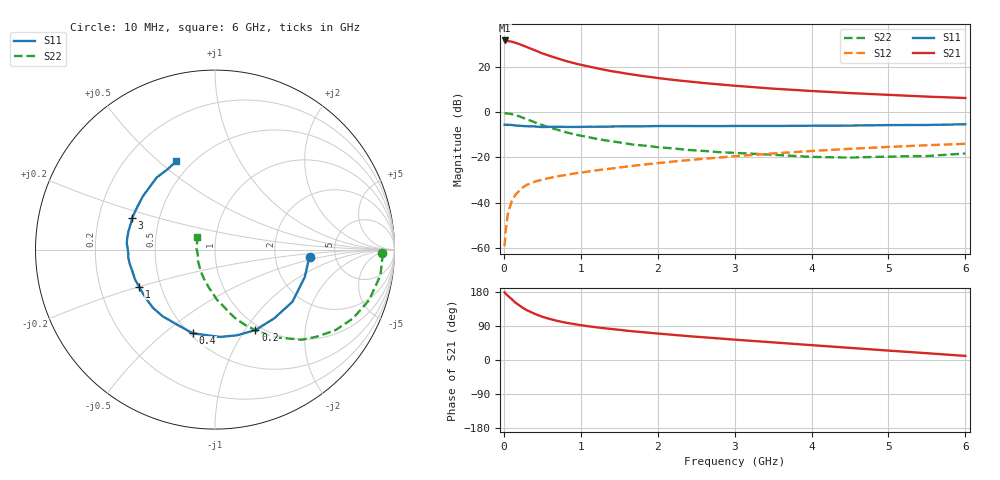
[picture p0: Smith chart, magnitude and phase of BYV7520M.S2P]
! SIEMENS Small Signal Semiconductors
! BFY420
! Si NPN RF SIEGET Grounded Emitter Transistor in MICRO-X
! VCE = 0.75 V  IC = 20 mA
! Common Emitter S-Parameters:  October  1996
# GHz  S  MA  R  50
!  f  S11  S21  S12  S22
! GHz  MAG  ANG  MAG  ANG  MAG  ANG  MAG  ANG
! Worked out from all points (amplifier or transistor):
!   36 points, 10 MHz to 6 GHz, reference 50 ohm
!   highest |S21| = 31.6 dB at 10 MHz (marker M1)
!   |S21| within 3 dB of that: start of sweep to 305.1 MHz
!   unconditionally stable (mu >= 1): 1.686 GHz to end of sweep
!   at 250 MHz: K = 0.32, MSG = 31.3 dB, |S12| = -33.2 dB
!   at 1.4 GHz: K = 0.94, MSG = 21.5 dB, |S12| = -24.9 dB
!   at 6 GHz: K = 1.10, MAG = 8.1 dB, |S12| = -14.0 dB
!   S11 on the Smith chart (normalised r, x): 10 MHz: 3.21, -0.35; 200 MHz: 0.93, -1.12; 400 MHz: 0.52, -0.63; 1 GHz: 0.38, -0.20; 3 GHz: 0.35, +0.17; 6 GHz: 0.41, +0.57
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0.01  0.5292 -4.2  38.08 178.7  0.0011 106.9  0.9319 -1.2
0.02  0.5235 -7.6  37.92 175.5  0.0021 92.7  0.9336 -3.1
0.1  0.5201 -34.0  35.88 161.0  0.0106 78.1  0.904 -18.1
0.15  0.5056 -49.2  33.84 151.4  0.015 71.0  0.8589 -26.5
0.2  0.5019 -63.3  31.8 144.4  0.0183 66.9  0.808 -33.7
0.25  0.4928 -75.7  29.42 137.1  0.022 62.4  0.7476 -40.4
0.3  0.4875 -86.6  27.18 131.2  0.0249 59.5  0.6979 -46.0
0.4  0.4826 -104.7  23.23 122.0  0.0291 55.5  0.5972 -55.1
0.5  0.4682 -118.0  19.77 114.1  0.0322 53.8  0.5167 -62.2
0.6  0.4724 -128.3  17.31 108.2  0.0354 52.3  0.4546 -67.9
0.7  0.4739 -136.7  15.27 103.0  0.0384 52.0  0.4055 -72.9
0.8  0.4711 -144.0  13.53 98.8  0.0408 51.2  0.3623 -77.0
1  0.4708 -154.1  11.08 92.0  0.046 51.9  0.3018 -83.8
1.1  0.4755 -159.4  10.18 89.0  0.0489 52.1  0.2798 -87.7
1.4  0.4807 -169.6  8.006 81.8  0.0568 52.2  0.2278 -96.0
1.6  0.4855 -175.0  7.033 77.3  0.0627 52.1  0.2016 -102.1
2.2  0.4931 172.3  5.14 66.4  0.0809 50.6  0.1581 -116.6
3  0.4942 158.8  3.821 53.7  0.1062 46.2  0.1261 -133.9
3.5  0.4942 150.5  3.293 46.5  0.1222 42.8  0.1144 -145.6
4.5  0.5042 136.1  2.629 32.0  0.1547 33.9  0.099 -168.8
5.5  0.5198 120.5  2.195 17.9  0.1856 24.0  0.1072 158.5
6  0.538 113.6  2.043 10.8  0.1999 18.8  0.122 145.0
